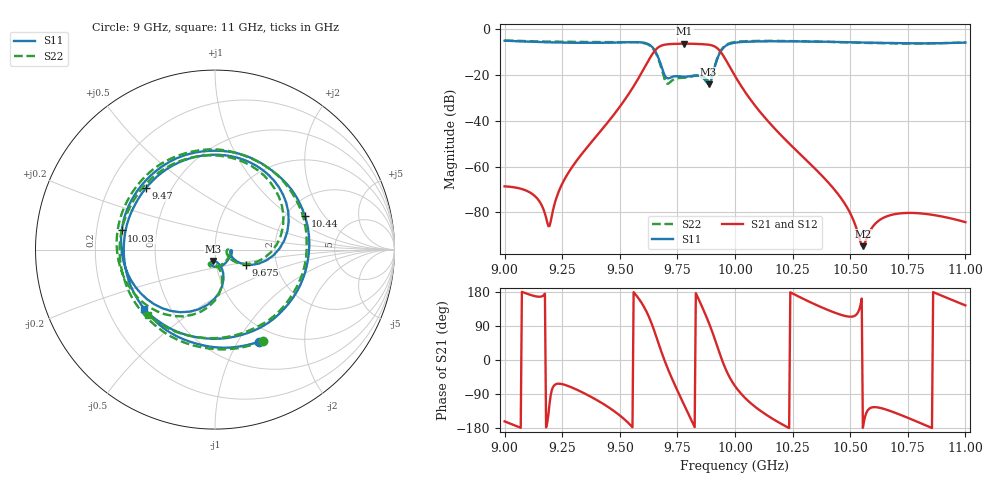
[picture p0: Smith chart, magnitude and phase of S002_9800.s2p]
# Hz S DB R 50
! Planar, S50180, , 20.4.1/1
! Date: 14.11.2021 18:36:29
! Data: Format (Calibration Info)
! Freq	S11:dB/Ang(--)	S21:dB/Ang(--)	S12:dB/Ang(--)	S22:dB/Ang(--)
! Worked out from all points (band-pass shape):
!   401 points, 9 GHz to 11 GHz, reference 50 ohm
!   highest |S21| = -6.21 dB at 9.78 GHz (marker M1); lowest = -94.8 dB at 10.55 GHz (marker M2)
!   |S21| within 3 dB of the highest: 9.653 GHz to 9.933 GHz (280 MHz wide, 2.86 % of centre)
!   lowest |S11| = -23.9 dB at 9.885 GHz (marker M3), VSWR 1.14, Z = 48.7 - j6.15 ohm
!   |S11| at or under -10 dB: 9.657 GHz to 9.936 GHz (279.2 MHz wide, 2.85 % of centre)
!   |S22| runs from -23.7 to -4.8 dB; largest |S21 - S12| = 0.00045
!   S11 on the Smith chart (normalised r, x): 9 GHz: 0.81, -1.23; 9.47 GHz: 0.36, +0.33; 9.675 GHz: 1.39, -0.24; 10.03 GHz: 0.31, +0.09; 10.44 GHz: 2.52, +1.31; 11 GHz: 0.36, -0.32
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9e9  -4.90 -64.4  -68.64 -162.0  -68.65 -162.0  -4.80 -62.5
9.2e9  -5.63 -123.8  -84.03 -92.9  -84.03 -92.9  -5.33 -119.7
9.335e9  -5.86 -168.6  -54.47 -84.6  -54.48 -84.6  -5.48 -162.6
9.47e9  -5.76 138.5  -37.80 -132.6  -37.81 -132.6  -5.52 146.4
9.585e9  -5.59 72.0  -20.64 159.5  -20.65 159.5  -5.69 79.9
9.635e9  -7.15 20.7  -11.77 101.2  -11.78 101.2  -7.44 26.2
9.67e9  -13.06 -22.4  -7.62 40.4  -7.62 40.3  -13.60 -22.1
9.675e9  -14.45 -26.0  -7.32 31.4  -7.33 31.4  -15.09 -26.9
9.705e9  -21.33 -10.8  -6.51 -17.9  -6.52 -18.0  -23.66 -11.8
9.78e9  -20.70 -32.4  -6.21 -119.5  -6.22 -119.6  -21.15 -46.3
9.83e9  -20.11 -75.4  -6.30 176.4  -6.31 176.4  -20.20 -89.0
9.885e9  -23.92 -98.7  -6.67 100.5  -6.67 100.4  -22.50 -104.0
9.93e9  -11.14 -91.1  -8.88 23.7  -8.88 23.7  -10.84 -90.7
1e10  -5.78 -173.1  -20.35 -68.7  -20.35 -68.7  -5.47 -165.2
1.0025e10  -5.50 168.4  -24.46 -88.0  -24.47 -88.0  -5.22 177.6
1.0155e10  -5.16 106.0  -41.46 -152.1  -41.46 -152.1  -4.97 118.5
1.0335e10  -5.31 48.3  -59.66 150.2  -59.67 150.2  -5.28 61.4
1.0435e10  -5.44 20.3  -70.48 124.4  -70.49 124.4  -5.50 32.4
1.05e10  -5.59 2.4  -80.37 114.2  -80.38 114.2  -5.69 13.9
1.0555e10  -5.71 -13.1  -94.82 -179.0  -94.83 -179.0  -5.85 -2.6
1.067e10  -5.92 -45.5  -81.38 -133.7  -81.39 -133.8  -6.08 -37.1
1.1e10  -5.75 -140.3  -84.31 144.1  -84.32 144.0  -5.66 -135.8
